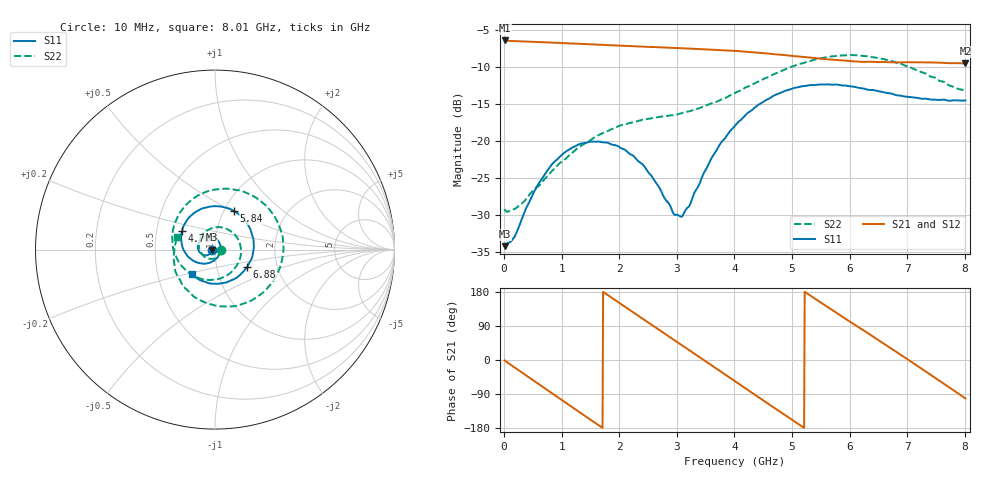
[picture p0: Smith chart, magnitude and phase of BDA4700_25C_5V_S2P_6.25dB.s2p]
!Agilent Technologies,E5071B,MY42404982,A.09.10
!Date: Mon Oct 20 13:29:04 2025
!Data & Calibration Information:
!Freq	S11:SOLT2(ON)	S21:SOLT2(ON)	S12:SOLT2(ON)	S22:SOLT2(ON)
# Hz S RI R 50
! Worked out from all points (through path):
!   801 points, 10 MHz to 8.01 GHz, reference 50 ohm
!   highest |S21| = -6.36 dB at 10 MHz (marker M1); lowest = -9.5 dB at 8.01 GHz (marker M2)
!   group delay of S21, straight-line fit = 284 ps
!   lowest |S11| = -34.2 dB at 10 MHz (marker M3), VSWR 1.04, Z = 48.1 - j0.0935 ohm
!   |S11| at or under -10 dB: start of sweep to end of sweep
!   |S22| runs from -29.6 to -8.3 dB; largest |S21 - S12| = 0.0037
!   S11 on the Smith chart (normalised r, x): 10 MHz: 0.96, -0.00; 4.78 GHz: 0.68, +0.15; 5.84 GHz: 1.11, +0.51; 6.88 GHz: 1.40, -0.28; 8.01 GHz: 0.74, -0.21
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1e7  -0.0194 -0.000971  0.4806 -0.0104  0.4807 -0.011  0.0345 -0.00283
3.3e8  -0.0247 -0.019  0.3866 -0.2733  0.3867 -0.2735  0.0227 -0.031
7.1e8  -0.0503 -0.0321  0.1197 -0.4514  0.1197 -0.4515  -0.0195 -0.0521
1.02e9  -0.079 -0.0215  -0.1387 -0.4399  -0.1391 -0.4402  -0.0652 -0.0338
1.35e9  -0.096 0.0102  -0.3583 -0.2813  -0.3586 -0.2814  -0.0899 0.0262
1.64e9  -0.0891 0.0443  -0.4457 -0.0628  -0.4458 -0.0628  -0.0662 0.0874
1.93e9  -0.063 0.0695  -0.4124 0.1664  -0.4125 0.1669  -0.000635 0.1232
2.32e9  -0.0152 0.0722  -0.2043 0.3869  -0.2044 0.3871  0.1015 0.0918
2.68e9  0.0213 0.0446  0.0685 0.4269  0.0684 0.4268  0.1451 -0.00808
2.95e9  0.0309 0.00874  0.2568 0.3422  0.2567 0.3417  0.12 -0.0901
3.09e9  0.0289 -0.0111  0.3324 0.266  0.3313 0.2666  0.0904 -0.1258
3.53e9  -0.0134 -0.0656  0.4154 -0.0471  0.4156 -0.0481  -0.0518 -0.1679
4.01e9  -0.1068 -0.0688  0.2282 -0.3387  0.2284 -0.3384  -0.1982 -0.0739
4.38e9  -0.1721 -0.00778  -0.0289 -0.3972  -0.0291 -0.3977  -0.239 0.0732
4.78e9  -0.184 0.1026  -0.2747 -0.2707  -0.2734 -0.2716  -0.1675 0.2426
5.35e9  -0.0626 0.2314  -0.357 0.0843  -0.3573 0.0835  0.1104 0.3336
5.84e9  0.104 0.2157  -0.1644 0.3124  -0.1633 0.3125  0.3378 0.1741
6.24e9  0.1971 0.1132  0.0689 0.3374  0.0723 0.3367  0.3724 -0.0622
6.68e9  0.2083 -0.0361  0.2823 0.1935  0.2831 0.193  0.2258 -0.2701
6.88e9  0.1791 -0.096  0.3304 0.0861  0.3309 0.0842  0.1181 -0.3136
7.48e9  0.018 -0.1903  0.2335 -0.2477  0.2336 -0.2487  -0.1809 -0.1997
8.01e9  -0.1305 -0.1367  -0.0668 -0.3293  -0.0665 -0.3295  -0.2091 0.0705
